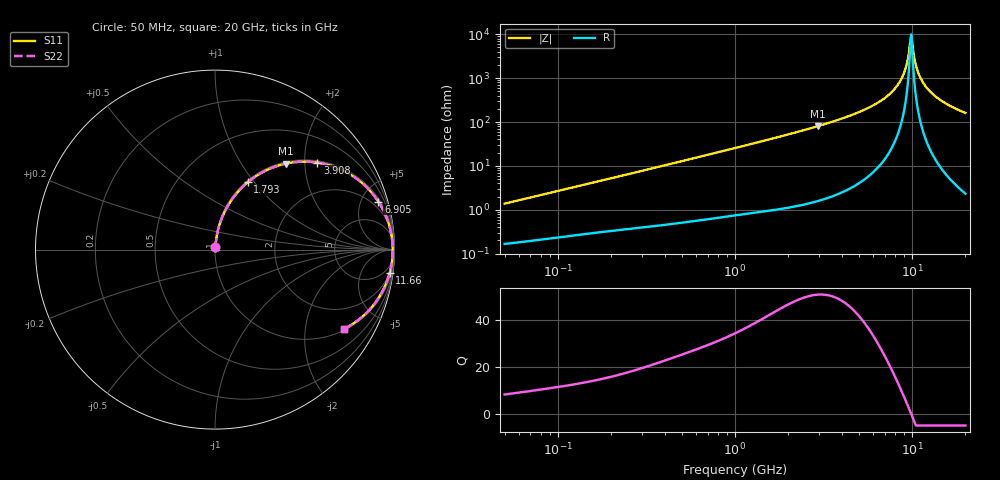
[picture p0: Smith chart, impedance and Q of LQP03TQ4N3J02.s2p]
!Murata Part Number: LQP03TQ4N3J02
!These Parameters are Measured in Series Mode Connection
!  o--[Z]--o
!Port1  Port2
!  o-------o
!Freq. Start=50[MHz] Stop=20[GHz], 401[Steps]
# Hz S RI R 50
!Freq.(Hz) S11(Real) S11(Imag) S21(Real) S21(Imag) S12(Real) S12(Imag) S22(Real) S22(Imag)
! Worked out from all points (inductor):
!   401 points, 50 MHz to 20 GHz, reference 50 ohm
!   read as one part in series: L = 4.32 nH near 51.52 MHz
!   highest Q = 50.9 at 2.94 GHz (marker M1), where L = 4.36 nH
!   self-resonance near 9.745 GHz
!   S11 on the Smith chart (normalised r, x): 50 MHz: 1.00, +0.03; 1.793 GHz: 1.02, +0.93; 3.908 GHz: 1.05, +2.31; 6.905 GHz: 1.26, +6.72; 11.66 GHz: 2, -15; 20 GHz: 1.05, -3.22
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5e7  0.00185 0.0136  0.9982 -0.0136  0.9982 -0.0136  0.00185 0.0136
1.364002e8  0.00402 0.0357  0.996 -0.0357  0.996 -0.0357  0.00402 0.0357
3.721004e8  0.0133 0.0938  0.9867 -0.0938  0.9867 -0.0938  0.0133 0.0938
1e9  0.067 0.2358  0.933 -0.2358  0.933 -0.2358  0.067 0.2358
1.793498e9  0.1829 0.3756  0.8171 -0.3756  0.8171 -0.3756  0.1829 0.3756
2.728004e9  0.3551 0.4688  0.6449 -0.4688  0.6449 -0.4688  0.3551 0.4688
2.940159e9  0.3955 0.4792  0.6045 -0.4792  0.6045 -0.4792  0.3955 0.4792
3.908127e9  0.5705 0.4849  0.4295 -0.4849  0.4295 -0.4849  0.5705 0.4849
5.433528e9  0.7843 0.3985  0.2157 -0.3985  0.2157 -0.3985  0.7843 0.3985
6.905011e9  0.91 0.2674  0.09 -0.2674  0.09 -0.2674  0.91 0.2674
7.442007e9  0.939 0.2166  0.061 -0.2166  0.061 -0.2166  0.939 0.2166
8.141811e9  0.9657 0.1511  0.0343 -0.1511  0.0343 -0.1511  0.9657 0.1511
8.774992e9  0.9807 0.0938  0.0193 -0.0938  0.0193 -0.0938  0.9807 0.0938
9.178299e9  0.9863 0.0586  0.0137 -0.0586  0.0137 -0.0586  0.9863 0.0586
9.745021e9  0.9899 0.0111  0.0101 -0.0111  0.0101 -0.0111  0.9899 0.0111
9.892087e9  0.99 -0.000853  0.00998 0.000853  0.00998 0.000853  0.99 -0.000853
1.004137e10  0.9899 -0.0128  0.0101 0.0128  0.0101 0.0128  0.9899 -0.0128
1.050288e10  0.9878 -0.0485  0.0122 0.0485  0.0122 0.0485  0.9878 -0.0485
1.082228e10  0.985 -0.0721  0.015 0.0721  0.015 0.0721  0.985 -0.0721
1.166392e10  0.973 -0.1304  0.027 0.1304  0.027 0.1304  0.973 -0.1304
1.438523e10  0.9043 -0.2797  0.0957 0.2797  0.0957 0.2797  0.9043 -0.2797
2e10  0.7187 -0.4425  0.2813 0.4425  0.2813 0.4425  0.7187 -0.4425
